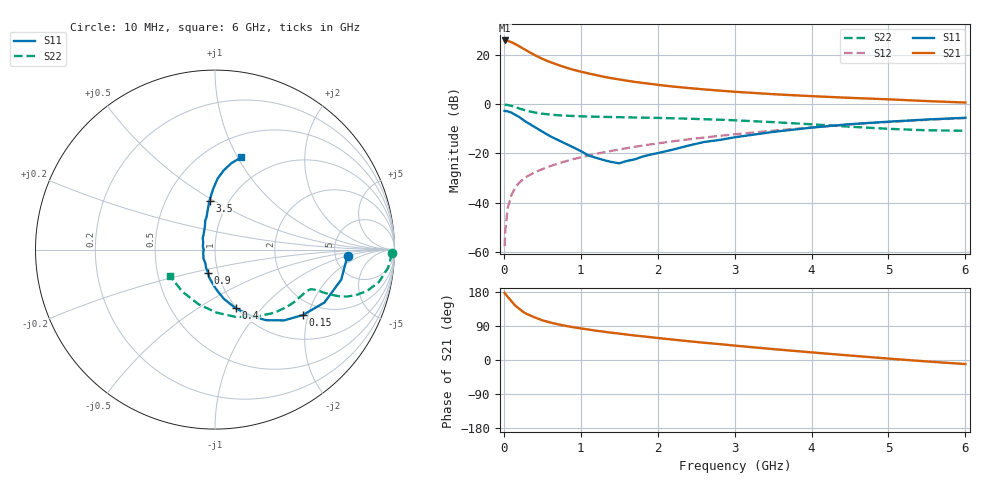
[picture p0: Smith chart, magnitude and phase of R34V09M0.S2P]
! SIEMENS Small Signal Semiconductors
! BFR181
! Si NPN RF Bipolar Junction Transistor in SOT23
! VCE = 4 V  IC = 9 mA
! Common Emitter S-Parameters:  May  1996
# GHz  S  MA  R  50
!  f  S11  S21  S12  S22
! GHz  MAG  ANG  MAG  ANG  MAG  ANG  MAG  ANG
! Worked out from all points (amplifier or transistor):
!   36 points, 10 MHz to 6 GHz, reference 50 ohm
!   highest |S21| = 26.0 dB at 10 MHz (marker M1)
!   |S21| within 3 dB of that: start of sweep to 234.5 MHz
!   unconditionally stable (mu >= 1): 849.3 MHz to 2.702 GHz
!   at 250 MHz: K = 0.57, MSG = 26.6 dB, |S12| = -30.5 dB
!   at 1.4 GHz: K = 1.06, MAG = 13.3 dB, |S12| = -18.9 dB
!   at 6 GHz: K = 0.86, MSG = 3.2 dB, |S12| = -5.6 dB
!   S11 on the Smith chart (normalised r, x): 10 MHz: 6.52, -1.00; 150 MHz: 1.59, -1.85; 400 MHz: 0.99, -0.73; 900 MHz: 0.90, -0.23; 3.5 GHz: 0.81, +0.48; 6 GHz: 0.72, +1.03
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0.01  0.7396 -2.7  19.98 177.0  0.0013 91.2  0.9863 -1.1
0.02  0.732 -5.6  19.91 174.2  0.0028 90.0  0.9816 -2.5
0.05  0.7228 -13.4  19.56 166.7  0.0077 80.9  0.9698 -6.0
0.1  0.6772 -25.8  18.43 154.8  0.0145 78.0  0.9309 -11.2
0.15  0.6102 -36.7  16.86 143.3  0.0205 73.5  0.8769 -15.3
0.2  0.5512 -45.7  15.23 135.0  0.0254 71.0  0.8249 -17.9
0.25  0.4863 -54.0  13.68 127.2  0.0297 68.7  0.7801 -19.6
0.3  0.4295 -60.5  12.32 121.2  0.034 68.4  0.7393 -20.6
0.4  0.3466 -70.6  10.11 112.5  0.0413 67.6  0.6832 -21.4
0.5  0.2793 -79.7  8.45 104.8  0.048 67.8  0.645 -21.6
0.6  0.2258 -87.5  7.287 99.2  0.0551 68.3  0.6199 -21.7
0.7  0.1895 -94.0  6.394 94.3  0.062 69.0  0.6011 -21.9
0.9  0.1341 -106.9  5.08 86.6  0.0768 68.9  0.5797 -22.4
1.1  0.0912 -126.6  4.265 80.4  0.0909 69.4  0.5654 -23.8
1.3  0.0734 -151.7  3.644 74.7  0.1061 69.1  0.5559 -25.3
1.6  0.0706 164.4  3.025 67.0  0.1286 68.3  0.5448 -28.3
2.2  0.1202 120.1  2.302 53.8  0.1772 65.2  0.5209 -35.9
2.6  0.1711 108.4  2.018 45.6  0.2112 62.4  0.4986 -41.9
3.5  0.2749 96.4  1.61 28.8  0.2918 54.7  0.4347 -59.4
4.5  0.3958 87.9  1.357 11.8  0.3892 43.9  0.351 -88.6
5.5  0.4918 79.1  1.166 -3.8  0.4834 31.2  0.2966 -127.9
6  0.5333 74.2  1.089 -10.8  0.5259 24.2  0.2905 -149.8
